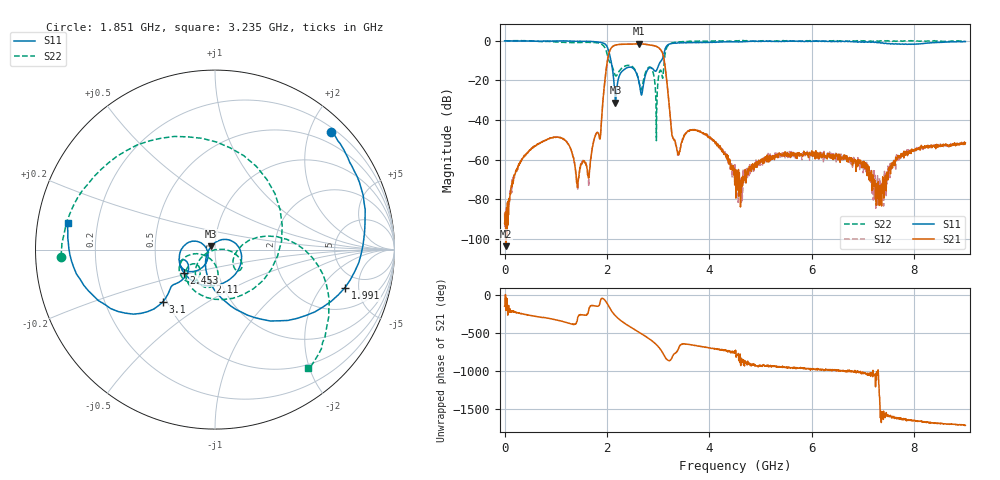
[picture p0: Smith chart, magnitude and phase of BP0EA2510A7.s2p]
!Agilent Technologies,E8358A,US40260310,A.06.04.32
!Agilent E8358A: A.06.04.32
!Date: Tuesday, September 01, 2020 10:48:09
!Correction: S11(Full 2 Port(1,2)) S21(Full 2 Port(1,2)) S12(Full 2 Port(1,2)) S22(Full 2 Port(1,2))
!S2P File: Measurements: S11, S21, S12, S22:
# Hz S  dB  R 50
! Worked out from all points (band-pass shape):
!   1601 points, 300 kHz to 9 GHz, reference 50 ohm
!   highest |S21| = -1.54 dB at 2.616 GHz (marker M1); lowest = -103.7 dB at 22.8 MHz (marker M2)
!   |S21| within 3 dB of the highest: 2.063 GHz to 3.049 GHz (985.8 MHz wide, 38.6 % of centre)
!   lowest |S11| = -31.3 dB at 2.166 GHz (marker M3), VSWR 1.06, Z = 47.9 + j1.67 ohm
!   |S11| at or under -10 dB: 2.077 GHz to 3.061 GHz (983.3 MHz wide, 38.3 % of centre)
!   |S22| runs from -50.5 to 0.2 dB; largest |S21 - S12| = 0.0042
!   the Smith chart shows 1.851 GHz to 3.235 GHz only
!   S11 on the Smith chart (normalised r, x): 1.851 GHz: 0.28, +2.37; 1.991 GHz: 3.55, -3.50; 2.11 GHz: 0.89, -0.33; 2.453 GHz: 0.69, -0.19; 3.1 GHz: 0.47, -0.33; 3.235 GHz: 0.09, +0.09
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300000  -0.04 180.0  -92.17 -144.6  -87.07 -12.9  -0.02 -0.2
2.279925e7  -0.03 179.0  -103.73 -109.3  -85.53 136.2  -0.03 -8.5
2.70291e8  -0.10 169.0  -63.23 128.2  -62.77 125.5  0.07 -90.3
6.30279e8  -0.22 154.7  -52.56 77.5  -52.53 81.2  -0.19 -167.6
1.114013e9  -0.08 130.5  -49.18 18.6  -49.10 17.8  -0.78 84.2
1.502125e9  -0.28 101.0  -62.44 102.8  -62.05 99.5  -0.80 -62.4
1.850863e9  -0.73 45.3  -48.60 -128.7  -48.81 -130.1  -1.30 -177.4
1.991484e9  -2.45 -16.4  -13.01 -96.0  -12.99 -95.5  -5.73 63.4
2.109605e9  -14.79 -99.3  -2.88 132.0  -2.92 132.1  -13.47 -140.5
2.165853e9  -31.25 140.5  -2.15 88.0  -2.14 88.0  -17.59 -140.7
2.452718e9  -13.31 -142.8  -1.68 -56.3  -1.69 -56.2  -12.52 -144.4
2.615838e9  -19.77 154.8  -1.54 -122.3  -1.53 -122.3  -19.66 -167.5
3.00395e9  -12.64 -137.4  -3.43 42.2  -3.43 42.1  -18.65 -12.1
3.099572e9  -7.67 -134.9  -7.58 -52.8  -7.57 -52.5  -16.13 10.0
3.234567e9  -1.57 169.6  -38.29 -136.3  -38.36 -137.2  -1.50 -51.9
3.386437e9  -1.06 126.5  -57.31 2.6  -57.73 4.9  -0.68 -83.2
3.91517e9  -0.88 16.4  -47.30 34.8  -47.33 36.3  -0.24 -123.9
4.50015e9  -0.57 -65.1  -65.57 -28.6  -61.83 -52.3  -0.15 -145.1
6.001975e9  -0.24 -159.9  -55.56 111.0  -56.86 110.5  -0.12 -169.0
7.5038e9  -1.37 77.7  -65.26 -144.7  -67.15 -153.3  -0.10 153.6
8.2519e9  -1.21 -68.7  -52.95 128.9  -53.24 126.2  -0.08 146.2
9e9  -0.38 -136.8  -51.55 89.7  -51.96 91.7  -0.47 143.7
